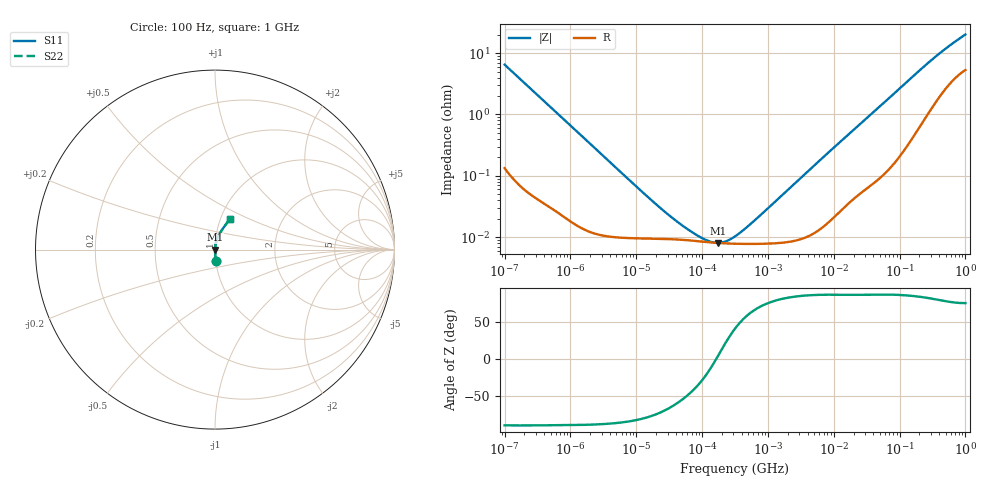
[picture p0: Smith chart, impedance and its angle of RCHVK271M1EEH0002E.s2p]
! RCHVK271M1EEH0002E  S-PARAMETER MODEL  (AEC-Q200 qualified)
! Model Generated by ELNA Corporation (http://www.ty-top.com)
! Version 1.0
! ELNA Control No. 240315
! Copyright (c) 2024 ELNA CO.,LTD. All Rights Reserved.
! Products Name : CONDUCTIVE POLYMER HYBRID ALUMINUM ELECTROLYTIC CAPACITORS
! Characteristics :
!  Capacitance  :  270uF  ,  Rated voltage  :  16V
!  Operating Temp. Range  :  -55 to +125 degC  ,  Endurance  :  4000hr at 125 degC
!  Dimension D  :  8mm  ,  Dimension L  :  10mm
! Frequency Range : 100Hz - 1GHz
! External Node Assignments :
!  1  o---| |---o  2
# MHz S RI R 50
!Freq[MHz].  S11 Real  S11 Imag  S21 Real  S21 Imag  S12 Real  S12 Imag  S22 Real  S22 Imag
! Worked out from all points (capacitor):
!   401 points, 100 Hz to 1 GHz, reference 50 ohm
!   read as one part in series: C = 245 uF near 108 Hz
!   lowest |Z| = 8.09 mohm at 172.8 kHz (marker M1)
!   series resonance near 164.2 kHz, so ESL is about 3.8 nH
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0.0001  0.00551 -0.0644  0.9945 0.0644  0.9945 0.0644  0.00551 -0.0644
0.000113  0.00441 -0.0572  0.9956 0.0572  0.9956 0.0572  0.00441 -0.0572
0.000309  0.000866 -0.0211  0.9991 0.0211  0.9991 0.0211  0.000866 -0.0211
0.001488  0.00016 -0.00446  0.9998 0.00446  0.9998 0.00446  0.00016 -0.00446
0.009495  9.67e-05 -0.0007  0.9999 0.0007  0.9999 0.0007  9.67e-05 -0.0007
0.022131  9.44e-05 -0.000299  0.9999 0.000299  0.9999 0.000299  9.44e-05 -0.000299
0.045709  9.14e-05 -0.00014  0.9999 0.00014  0.9999 0.00014  9.14e-05 -0.00014
0.063096  8.9e-05 -9.56e-05  0.9999 9.56e-05  0.9999 9.56e-05  8.9e-05 -9.56e-05
0.087096  8.62e-05 -6e-05  0.9999 6e-05  0.9999 6e-05  8.62e-05 -6e-05
0.102329  8.47e-05 -4.41e-05  0.9999 4.41e-05  0.9999 4.41e-05  8.47e-05 -4.41e-05
0.172783  8.07e-05 4.74e-06  0.9999 -4.74e-06  0.9999 -4.74e-06  8.07e-05 4.74e-06
0.280221  7.87e-05 5.32e-05  0.9999 -5.32e-05  0.9999 -5.32e-05  7.87e-05 5.32e-05
0.316228  7.84e-05 6.7e-05  0.9999 -6.7e-05  0.9999 -6.7e-05  7.84e-05 6.7e-05
0.419276  7.79e-05 0.000103  0.9999 -0.000103  0.9999 -0.000103  7.79e-05 0.000103
0.627336  7.79e-05 0.000171  0.9999 -0.000171  0.9999 -0.000171  7.79e-05 0.000171
4.704354  0.000113 0.00137  0.9999 -0.00137  0.9999 -0.00137  0.000113 0.00137
69.9842  0.00164 0.0186  0.9984 -0.0186  0.9984 -0.0186  0.00164 0.0186
163.1173  0.00614 0.042  0.9939 -0.042  0.9939 -0.042  0.00614 0.042
336.8992  0.0209 0.08  0.9791 -0.08  0.9791 -0.08  0.0209 0.08
592.2431  0.0468 0.1214  0.9532 -0.1214  0.9532 -0.1214  0.0468 0.1214
922.5714  0.0756 0.1608  0.9244 -0.1608  0.9244 -0.1608  0.0756 0.1608
1000  0.0815 0.1691  0.9185 -0.1691  0.9185 -0.1691  0.0815 0.1691
